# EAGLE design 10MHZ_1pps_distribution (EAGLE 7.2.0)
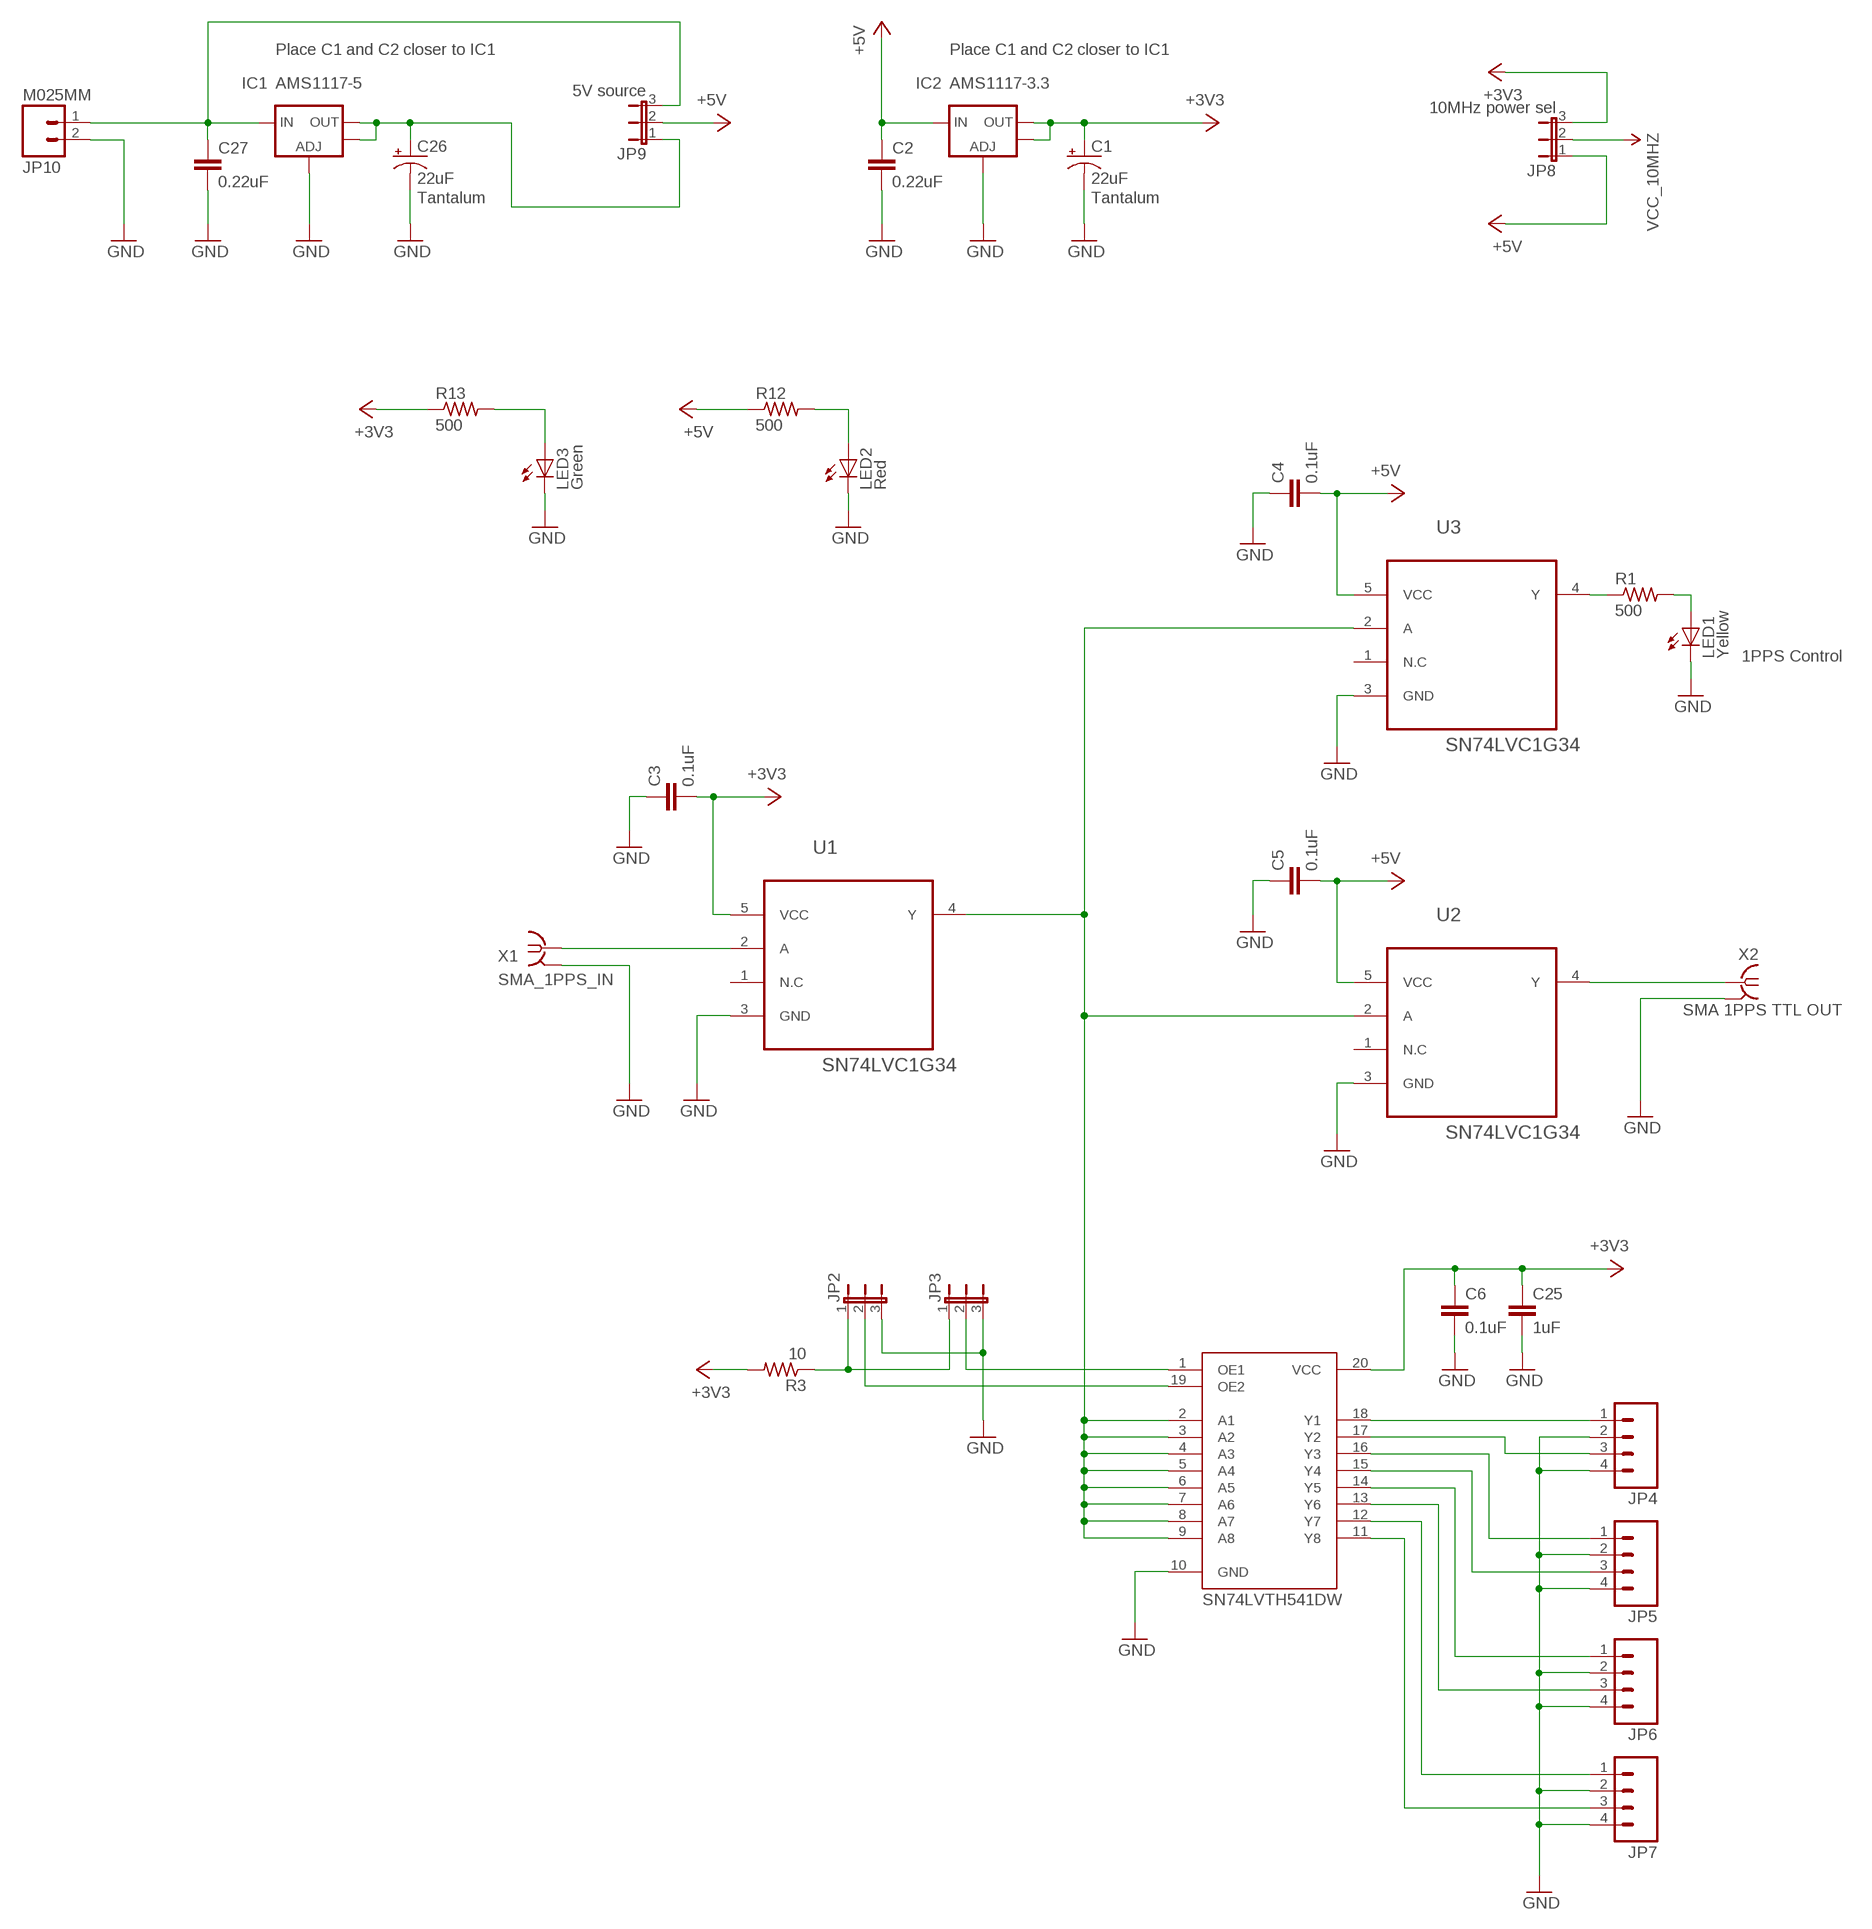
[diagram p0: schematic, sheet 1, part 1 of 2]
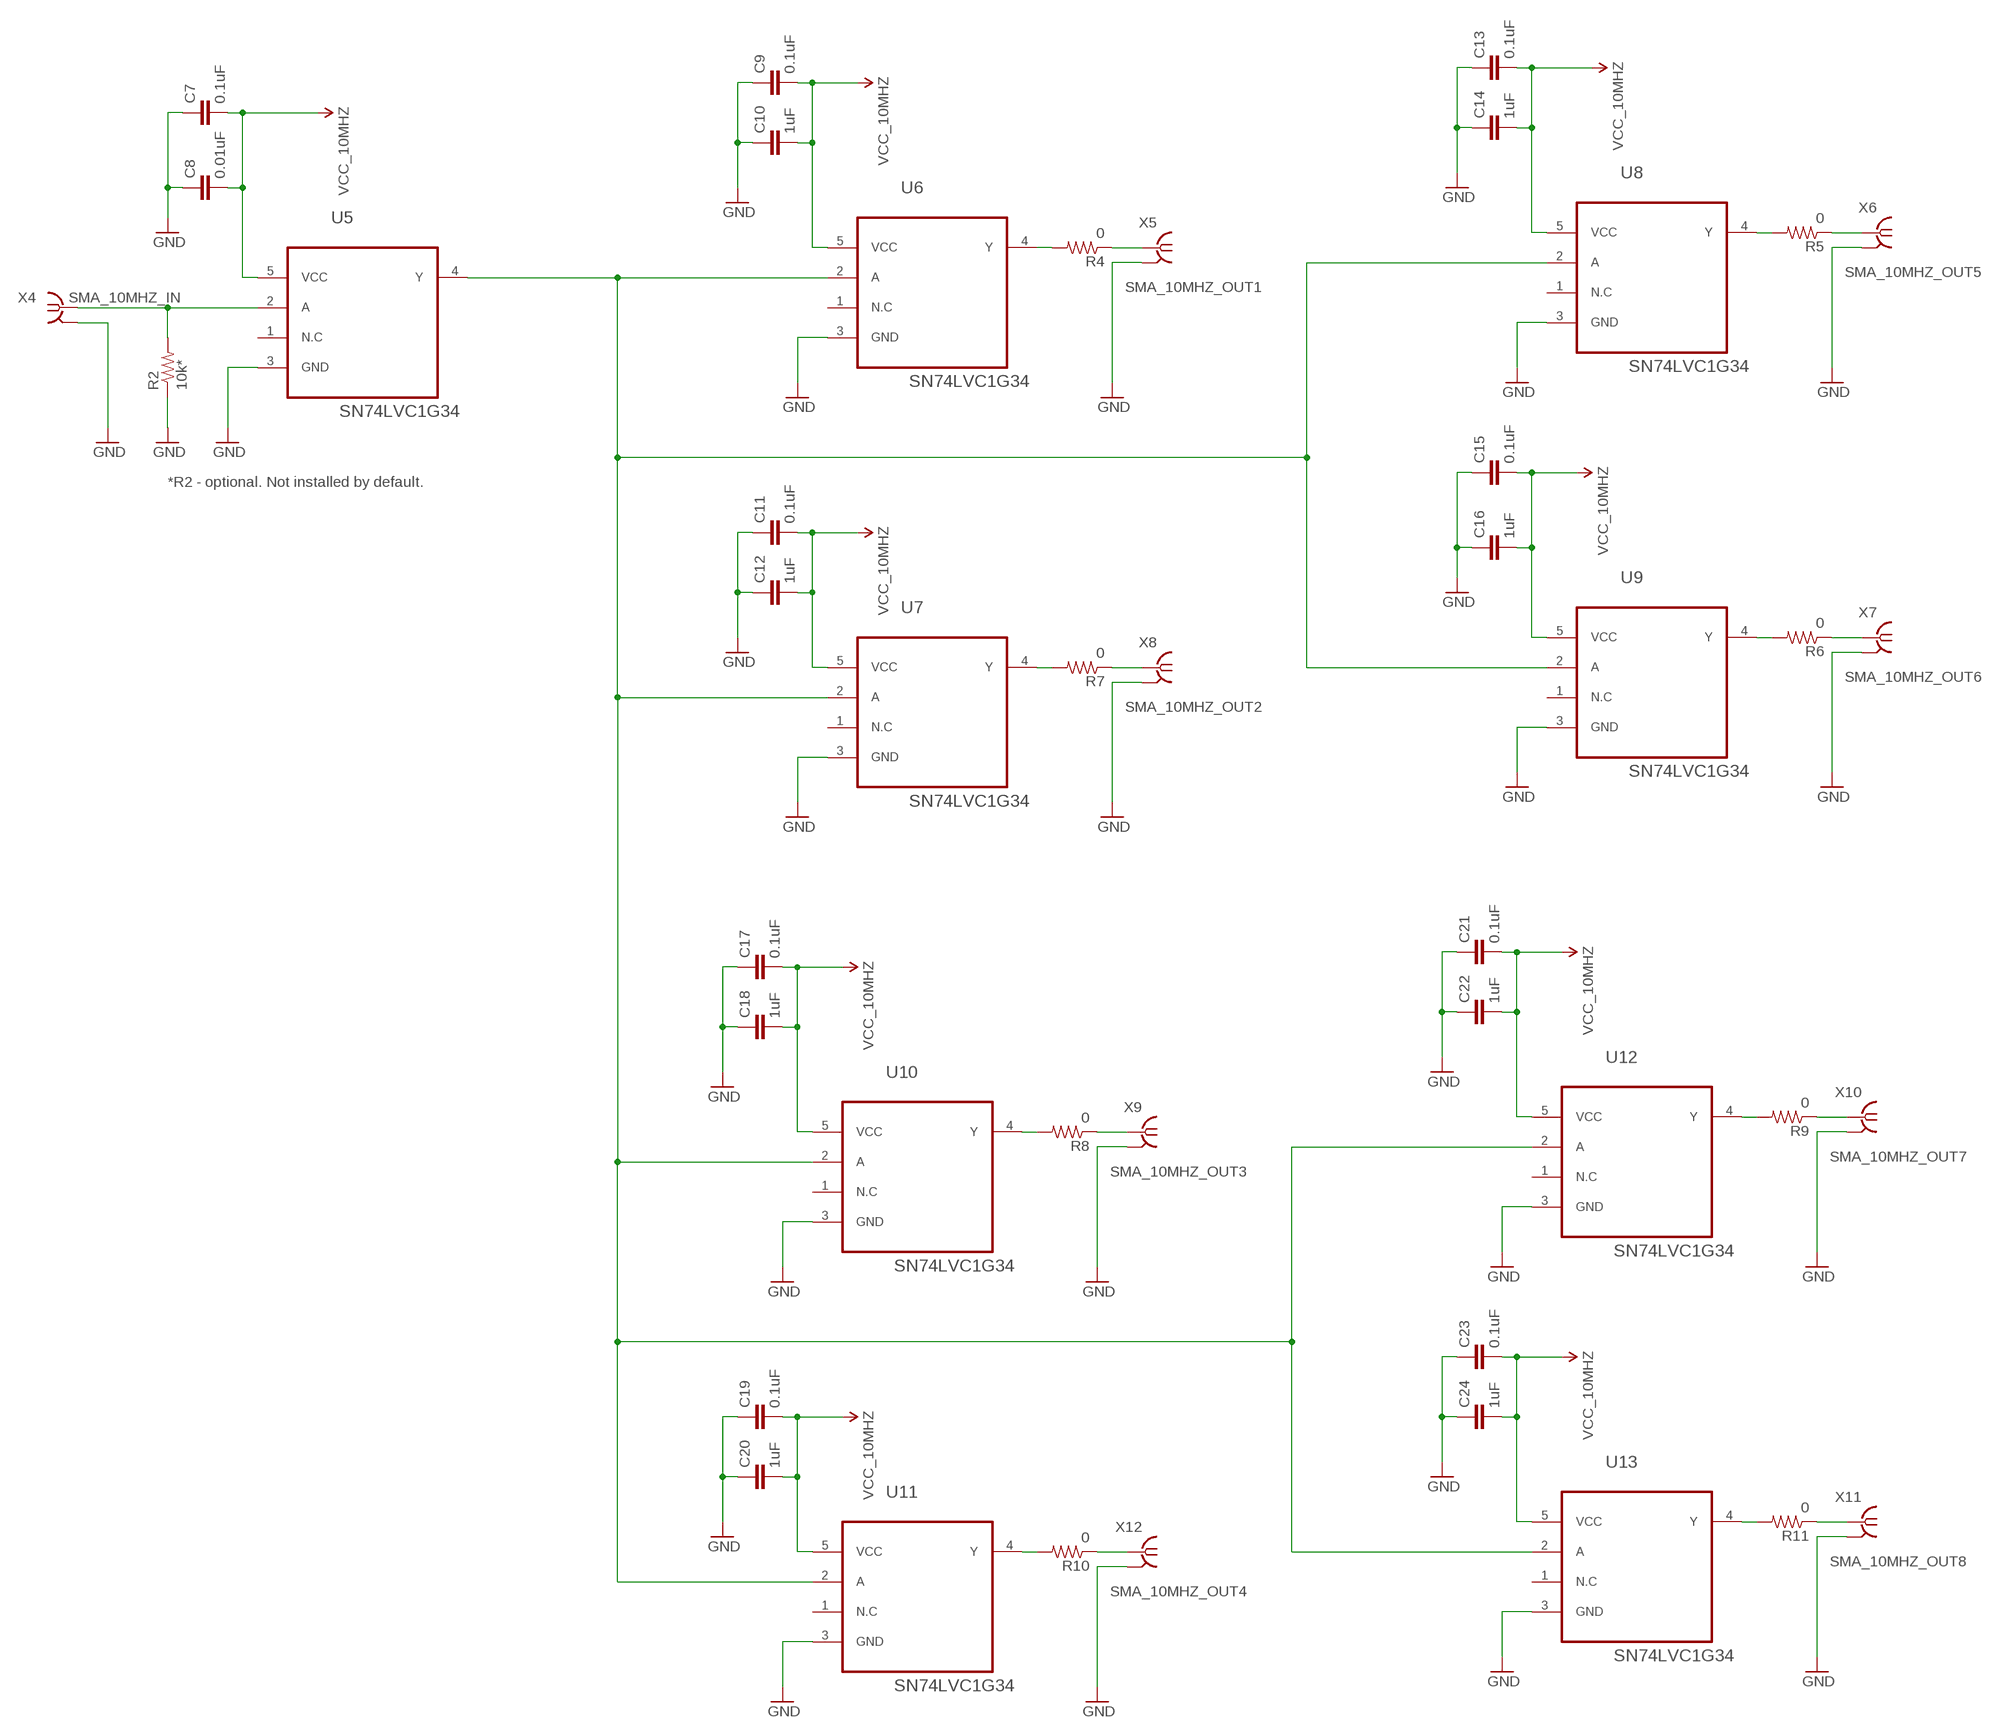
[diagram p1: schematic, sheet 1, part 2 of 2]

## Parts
C1  22uF  CPOL-USD/7343-31W  [D/7343-31W]
C2  0.22uF  C-EUC0805  [C0805]
C3  0.1uF  C-EUC0805  [C0805]
C4  0.1uF  C-EUC0805  [C0805]
C5  0.1uF  C-EUC0805  [C0805]
C6  0.1uF  C-EUC0805  [C0805]
C7  0.1uF  C-EUC0805  [C0805]
C8  0.01uF  C-EUC0805  [C0805]
C9  0.1uF  C-EUC0805  [C0805]
C10  1uF  C-EUC0805  [C0805]
C11  0.1uF  C-EUC0805  [C0805]
C12  1uF  C-EUC0805  [C0805]
C13  0.1uF  C-EUC0805  [C0805]
C14  1uF  C-EUC0805  [C0805]
C15  0.1uF  C-EUC0805  [C0805]
C16  1uF  C-EUC0805  [C0805]
C17  0.1uF  C-EUC0805  [C0805]
C18  1uF  C-EUC0805  [C0805]
C19  0.1uF  C-EUC0805  [C0805]
C20  1uF  C-EUC0805  [C0805]
C21  0.1uF  C-EUC0805  [C0805]
C22  1uF  C-EUC0805  [C0805]
C23  0.1uF  C-EUC0805  [C0805]
C24  1uF  C-EUC0805  [C0805]
C25  1uF  C-EUC0805  [C0805]
C26  22uF  CPOL-USD/7343-31W  [D/7343-31W]
C27  0.22uF  C-EUC0805  [C0805]
IC1  AMS1117-5  LD117AS12TR  [SOT223]
IC2  AMS1117-3.3  LD117AS12TR  [SOT223]
JP2  JP2E  [JP2]
JP3  JP2E  [JP2]
JP4  M04LOCK  [1X04_LOCK]
JP5  M04LOCK  [1X04_LOCK]
JP6  M04LOCK  [1X04_LOCK]
JP7  M04LOCK  [1X04_LOCK]
JP8  10MHz power sel  JP2E  [JP2]
JP9  5V source  JP2E  [JP2]
JP10  M025MM  [SCREWTERMINAL-5MM-2]
LED1  Yellow  LEDSML0805  [SML0805]
LED2  Red  LEDSML0805  [SML0805]
LED3  Green  LEDSML0805  [SML0805]
R1  500  R-US_R0805  [R0805]
R2  10k*  R-US_R0805  [R0805]
R3  10  R-US_R0805  [R0805]
R4  0  R-US_R0805  [R0805]
R5  0  R-US_R0805  [R0805]
R6  0  R-US_R0805  [R0805]
R7  0  R-US_R0805  [R0805]
R8  0  R-US_R0805  [R0805]
R9  0  R-US_R0805  [R0805]
R10  0  R-US_R0805  [R0805]
R11  0  R-US_R0805  [R0805]
R12  500  R-US_R0805  [R0805]
R13  500  R-US_R0805  [R0805]
U1  SN74LVC1G34  SN74LVC1G07DCK6  [SOT65P210X110-5N]
U2  SN74LVC1G34  SN74LVC1G07DCK6  [SOT65P210X110-5N]
U3  SN74LVC1G34  SN74LVC1G07DCK6  [SOT65P210X110-5N]
U4  SN74LVTH541DW  [SOIC127P1030X265-20N]
U5  SN74LVC1G34  SN74LVC1G07DCK6  [SOT65P210X110-5N]
U6  SN74LVC1G34  SN74LVC1G07DCK6  [SOT65P210X110-5N]
U7  SN74LVC1G34  SN74LVC1G07DCK6  [SOT65P210X110-5N]
U8  SN74LVC1G34  SN74LVC1G07DCK6  [SOT65P210X110-5N]
U9  SN74LVC1G34  SN74LVC1G07DCK6  [SOT65P210X110-5N]
U10  SN74LVC1G34  SN74LVC1G07DCK6  [SOT65P210X110-5N]
U11  SN74LVC1G34  SN74LVC1G07DCK6  [SOT65P210X110-5N]
U12  SN74LVC1G34  SN74LVC1G07DCK6  [SOT65P210X110-5N]
U13  SN74LVC1G34  SN74LVC1G07DCK6  [SOT65P210X110-5N]
X1  SMA_1PPS_IN  SMA-142-0701-801/806  [J502-ND-142-0701-801/806]
X2  SMA 1PPS TTL OUT  SMA-142-0701-801/806  [J502-ND-142-0701-801/806]
X4  SMA_10MHZ_IN  SMA-142-0701-801/806  [J502-ND-142-0701-801/806]
X5  SMA_10MHZ_OUT1  SMA-142-0701-801/806  [J502-ND-142-0701-801/806]
X6  SMA_10MHZ_OUT5  SMA-142-0701-801/806  [J502-ND-142-0701-801/806]
X7  SMA_10MHZ_OUT6  SMA-142-0701-801/806  [J502-ND-142-0701-801/806]
X8  SMA_10MHZ_OUT2  SMA-142-0701-801/806  [J502-ND-142-0701-801/806]
X9  SMA_10MHZ_OUT3  SMA-142-0701-801/806  [J502-ND-142-0701-801/806]
X10  SMA_10MHZ_OUT7  SMA-142-0701-801/806  [J502-ND-142-0701-801/806]
X11  SMA_10MHZ_OUT8  SMA-142-0701-801/806  [J502-ND-142-0701-801/806]
X12  SMA_10MHZ_OUT4  SMA-142-0701-801/806  [J502-ND-142-0701-801/806]

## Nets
10MHZ_ROUTE1: U5.4(Y) U6.2(A) U7.2(A) U8.2(A) U9.2(A) U10.2(A) U11.2(A) U12.2(A) U13.2(A)
+3V3: C1.+ C3.2 C6.1 C25.1 IC2.2(OUT) IC2.4(OUT1) JP8.3 R3.2 R13.1 U1.5(VCC) U4.20(VCC)
+5V: C2.1 C4.2 C5.2 IC2.3(IN) JP8.1 JP9.2 R12.1 U2.5(VCC) U3.5(VCC)
GND: C1.- C2.2 C3.1 C4.1 C5.1 C6.2 C7.1 C8.1 C9.1 C10.1 C11.1 C12.1 C13.1 C14.1 C15.1 C16.1 C17.1 C18.1 C19.1 C20.1 C21.1 C22.1 C23.1 C24.1 C25.2 C26.- C27.2 IC1.1(ADJ) IC2.1(ADJ) JP2.3 JP3.3 JP4.2 JP4.4 JP5.2 JP5.4 JP6.2 JP6.4 JP7.2 JP7.4 JP10.2 LED1.C LED2.C LED3.C R2.1 U1.3(GND) U2.3(GND) U3.3(GND) U4.10(GND) U5.3(GND) U6.3(GND) U7.3(GND) U8.3(GND) U9.3(GND) U10.3(GND) U11.3(GND) U12.3(GND) U13.3(GND) X1.G@1(GND) X2.G@1(GND) X4.G@1(GND) X5.G@1(GND) X6.G@1(GND) X7.G@1(GND) X8.G@1(GND) X9.G@1(GND) X10.G@1(GND) X11.G@1(GND) X12.G@1(GND)
N$1: U1.2(A) X1.1
N$2: R1.1 U3.4(Y)
N$3: LED1.A R1.2
N$4: U1.4(Y) U2.2(A) U3.2(A) U4.2(A1) U4.3(A2) U4.4(A3) U4.5(A4) U4.6(A5) U4.7(A6) U4.8(A7) U4.9(A8)
N$5: U2.4(Y) X2.1
N$6: JP3.2 U4.1(OE1)
N$7: JP2.2 U4.19(OE2)
N$8: LED2.A R12.2
N$9: LED3.A R13.2
N$10: JP2.1 JP3.1 R3.1
N$14: R2.2 U5.2(A) X4.1
N$15: R8.2 U10.4(Y)
N$16: R10.2 U11.4(Y)
N$17: R4.1 X5.1
N$18: R9.2 U12.4(Y)
N$19: R7.2 U7.4(Y)
N$20: R11.2 U13.4(Y)
N$21: R5.2 U8.4(Y)
N$23: R6.2 U9.4(Y)
N$27: C27.1 IC1.3(IN) JP9.3 JP10.1
N$28: R4.2 U6.4(Y)
N$29: C26.+ IC1.2(OUT) IC1.4(OUT1) JP9.1
N$30: R5.1 X6.1
N$31: R7.1 X8.1
N$32: R6.1 X7.1
N$33: R8.1 X9.1
N$34: R9.1 X10.1
N$35: R10.1 X12.1
N$36: R11.1 X11.1
PPS_OUT_Y1: JP4.1 U4.18(Y1)
PPS_OUT_Y2: JP4.3 U4.17(Y2)
PPS_OUT_Y3: JP5.1 U4.16(Y3)
PPS_OUT_Y4: JP5.3 U4.15(Y4)
PPS_OUT_Y5: JP6.1 U4.14(Y5)
PPS_OUT_Y6: JP6.3 U4.13(Y6)
PPS_OUT_Y7: JP7.1 U4.12(Y7)
PPS_OUT_Y8: JP7.3 U4.11(Y8)
VCC_10MHZ: C7.2 C8.2 C9.2 C10.2 C11.2 C12.2 C13.2 C14.2 C15.2 C16.2 C17.2 C18.2 C19.2 C20.2 C21.2 C22.2 C23.2 C24.2 JP8.2 U5.5(VCC) U6.5(VCC) U7.5(VCC) U8.5(VCC) U9.5(VCC) U10.5(VCC) U11.5(VCC) U12.5(VCC) U13.5(VCC)
Unconnected: U1.1(N.C) U2.1(N.C) U3.1(N.C) U5.1(N.C) U6.1(N.C) U7.1(N.C) U8.1(N.C) U9.1(N.C) U10.1(N.C) U11.1(N.C) U12.1(N.C) U13.1(N.C)

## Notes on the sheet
- Place C1 and C2 closer to IC1 | Place C1 and C2 closer to IC1
- Tantalum | Tantalum
- *R2 - optional. Not installed by default.
- 1PPS Control

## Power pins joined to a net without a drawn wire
GND: X1.G@2(GND) X1.G@3(GND) X1.G@4(GND) X2.G@2(GND) X2.G@3(GND) X2.G@4(GND) X4.G@2(GND) X4.G@3(GND) X4.G@4(GND) X5.G@2(GND) X5.G@3(GND) X5.G@4(GND) X6.G@2(GND) X6.G@3(GND) X6.G@4(GND) X7.G@2(GND) X7.G@3(GND) X7.G@4(GND) X8.G@2(GND) X8.G@3(GND) X8.G@4(GND) X9.G@2(GND) X9.G@3(GND) X9.G@4(GND) X10.G@2(GND) X10.G@3(GND) X10.G@4(GND) X11.G@2(GND) X11.G@3(GND) X11.G@4(GND) X12.G@2(GND) X12.G@3(GND) X12.G@4(GND)

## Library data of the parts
C1 C26 = resistor:CPOL-US: POLARIZED CAPACITOR, American symbol
C2-C25 C27 = resistor:C-EU: CAPACITOR, European symbol
IC1 IC2 = v-reg:LD117A?*: Low drop fixed and adjustable positive voltage regulators 1 A Source: http://www.st.com/stonline/products/literature/ds/7194/ld1117axx.pdf
JP2 JP3 JP8 JP9 = jumper:JP2E: JUMPER
JP4-JP7 = SparkFun-Connectors:M04: Header 4 Standard 4-pin 0.1" header. Use with straight break away headers (SKU : PRT-00116), right angle break away headers (PRT-00553), swiss pins (PRT-00743), machine pins (PRT-00117), and female headers (PRT-00115). Molex polarized connector foot print use with SKU : PRT-08231 with associated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
JP10 = SparkFun-Connectors:M02: Standard 2-pin 0.1" header. Use with
LED1-LED3 = led:LED: LED
R1 R12 R13 = rcl:R-US_: RESISTOR, American symbol
R2-R11 = adafruit:R-US_: RESISTOR, American symbol
U1-U3 U5-U13 = Texas Instruments_By_element14_Batch_1:SN74LVC1G07DCK6: BUFFER; MPN: SN74LVC1G07DCK6; OC_FARNELL: 1236609; OC_NEWARK: 13M2906; PACKAGE: SC-70-5; SUPPLIER: Texas Instruments
U4 = Texas Instruments_By_element14_Batch_1:SN74LVTH541DW: ABT OCTAL buffer/driver with 3-state outputs; MPN: SN74LVTH541DW; PACKAGE: SOIC-20; SUPPLIER: Texas Instruments
X1 X2 X4-X12 = con-coax:SMA-: SMA 50 Ohm End Launch Jack Receptacle - Round Contact Johnson Components Source: www.johnsoncomponents.com .. J502-ND.pdf

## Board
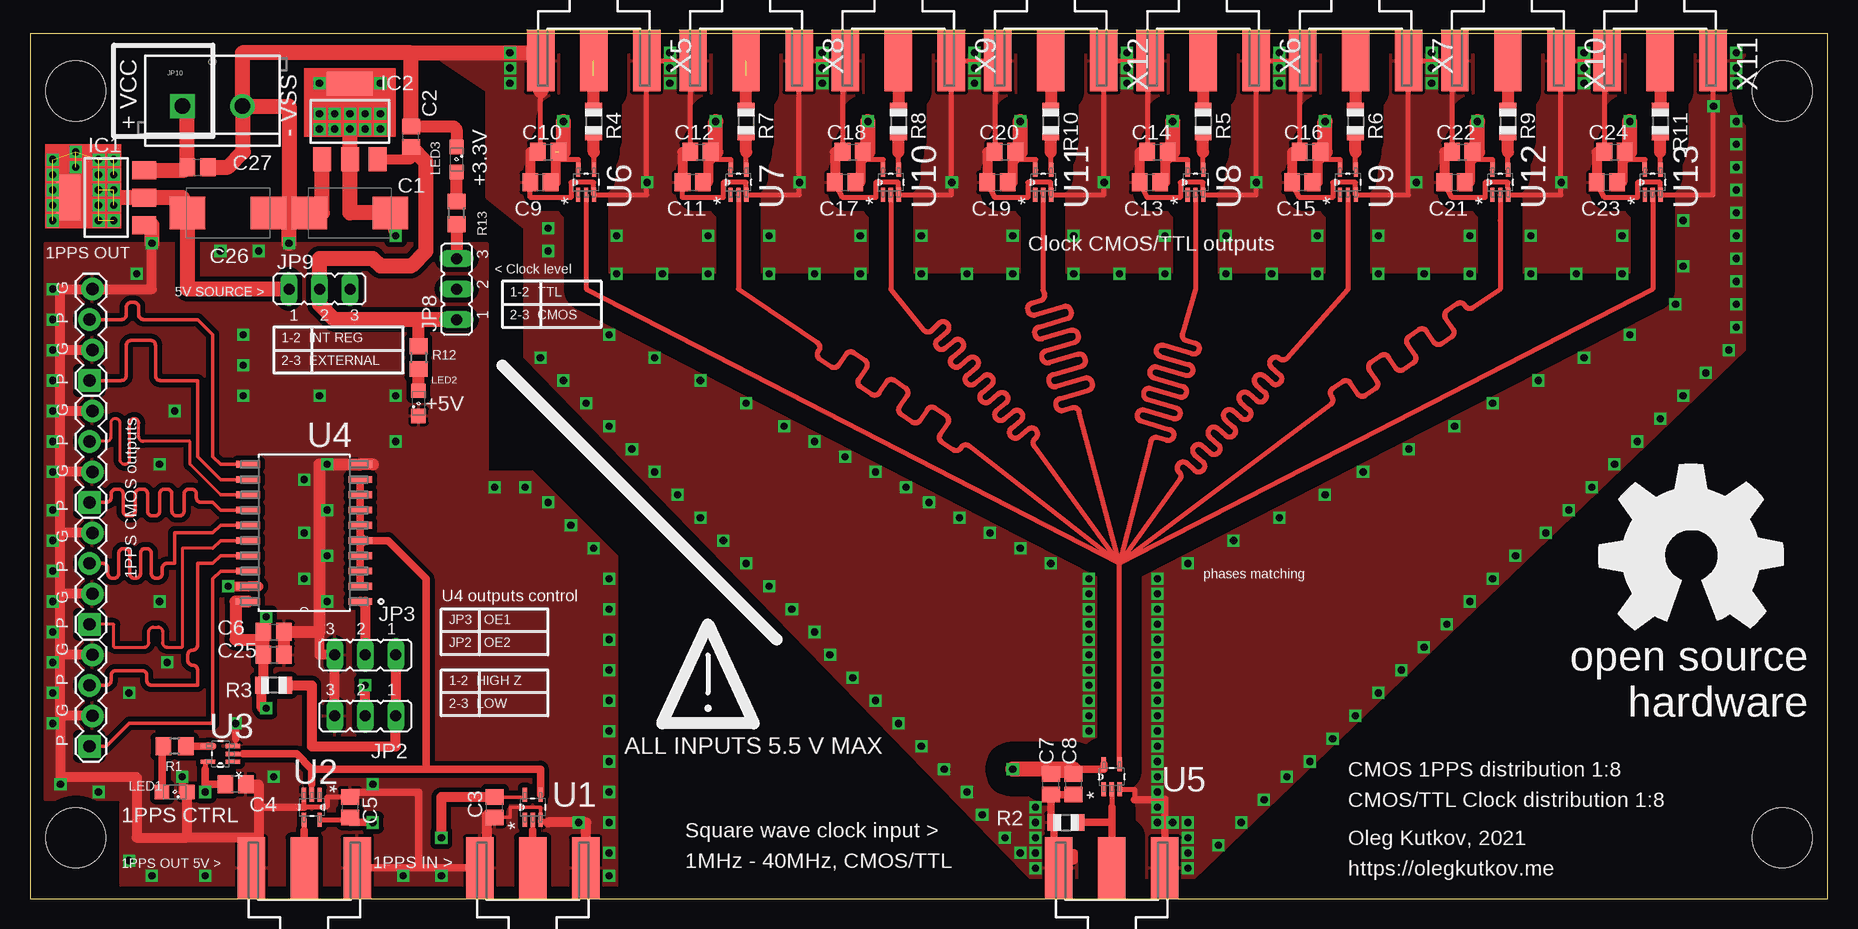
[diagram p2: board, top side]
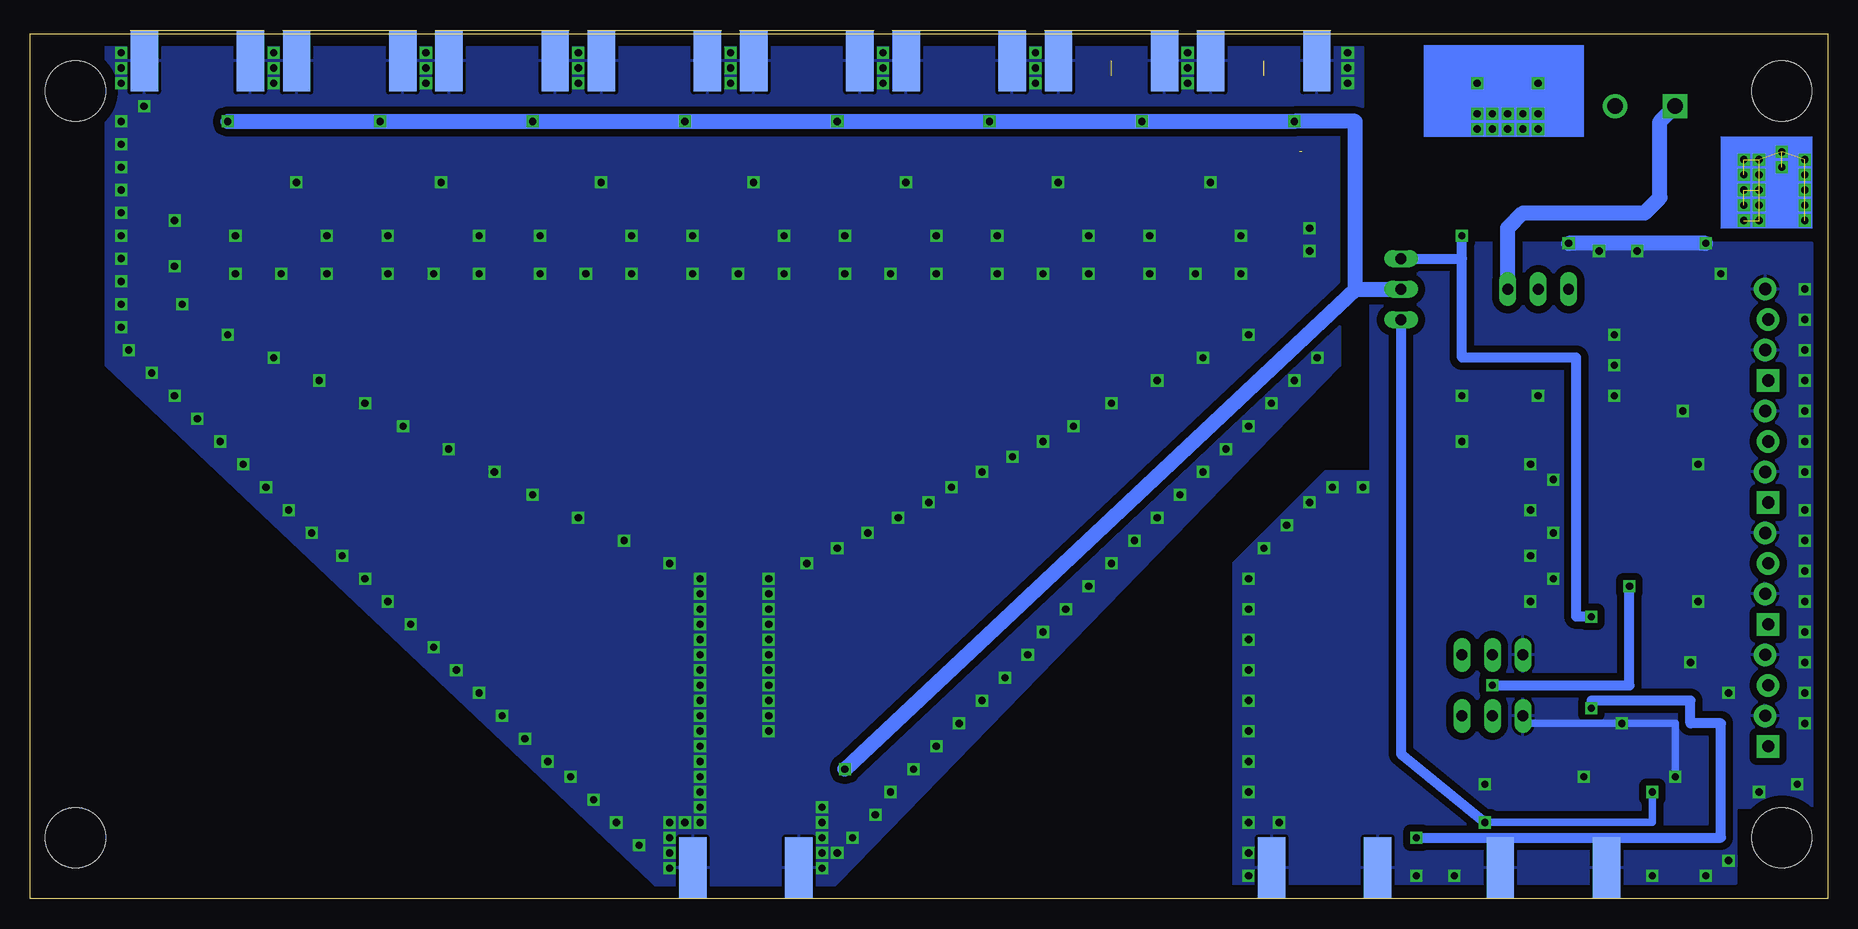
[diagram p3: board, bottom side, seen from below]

Size 149.84 x 72.39 mm. Coordinates in mm from the lower left corner, seen from the top.
Outline: 0,0 149.84,0 149.84,72.06 0,72.06 0,0
Copper layers (1*16): Top 0.035mm / dielectric 1.5mm / Bottom 0.035mm
Design rules "default": minimum track width 10mil, minimum drill 24mil, track to track 8mil, track to pad 8mil, pad to pad 8mil, via to via 8mil, smd to smd 8mil, copper to edge 40mil, drill to drill 8mil, minimum pad ring 10mil, minimum via ring 8mil, stop-mask expansion 4mil, vias tented up to drill 0mil, thermal gap 10mil
Holes 5 mm at 3.81,67.31 146.05,67.31 146.05,5.08 3.81,5.08

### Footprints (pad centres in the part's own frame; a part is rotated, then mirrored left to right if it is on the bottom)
D/7343-31W = smd 2.95 x 2.7: + 3.375,0; - -3.375,0
C0805 = smd 1.3 x 1.5: 1 -0.85,0; 2 0.85,0
SOT223 = smd 1.5 x 2: 1 -2.3,-3.15; 2 0,-3.15; 3 2.3,-3.15 | smd 3.8 x 2: 4 0,3.15
JP2 = drill 0.914 long: 1 -2.54,0; 2 0,0; 3 2.54,0
1X04_LOCK = drill 1.016 pad 1.88 square: 1 0,0.127 | drill 1.016 pad 1.88: 2 2.54,-0.127; 3 5.08,0.127; 4 7.62,-0.127
SCREWTERMINAL-5MM-2 = drill 1.3 pad 2.032 square: 1 0,0 | drill 1.3 pad 2.032: 2 5,0
SML0805 = smd 1.2 x 1.2: A 1.05,0; C -1.05,0
R0805 = smd 1.3 x 1.5: 1 -0.95,0; 2 0.95,0
R0805' = smd 1.1 x 1.4: 1 -1,0; 2 1,0
SOT65P210X110-5N = smd 1.168 x 0.356: 1 -1.041,0.66; 2 -1.041,0; 3 -1.041,-0.66; 4 1.041,-0.66; 5 1.041,0.66
SOIC127P1030X265-20N = smd 1.981 x 0.559: 1 -4.674,5.715; 2 -4.674,4.445; 3 -4.674,3.175; 4 -4.674,1.905; 5 -4.674,0.635; 6 -4.674,-0.635; 7 -4.674,-1.905; 8 -4.674,-3.175; 9 -4.674,-4.445; 10 -4.674,-5.715; 11 4.674,-5.715; 12 4.674,-4.445; 13 4.674,-3.175; 14 4.674,-1.905; 15 4.674,-0.635; 16 4.674,0.635; 17 4.674,1.905; 18 4.674,3.175; 19 4.674,4.445; 20 4.674,5.715
J502-ND-142-0701-801/806 = smd 5.08 x 2.286: 1 2.565,0; G@1 2.565,4.42; G@2 2.565,-4.42 | smd 5.08 x 2.286 bottom: G@3 2.565,4.42; G@4 2.565,-4.42

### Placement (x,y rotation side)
C1  26.67,57.15 0 top
C2  31.75,63.5 90 top
C3  38.73,7.62 90 top
C4  17.14,9.53 180 top
C5  26.67,7.62 270 top
C6  20.32,22.22 0 top
C7  85.09,9.53 90 top
C8  87,9.53 90 top
C9  42.55,59.69 0 top
C10  43.18,62.23 0 top
C11  55.24,59.69 0 top
C12  55.88,62.23 0 top
C13  93.34,59.69 0 top
C14  93.98,62.23 0 top
C15  106.05,59.69 0 top
C16  106.68,62.23 0 top
C17  67.94,59.69 0 top
C18  68.58,62.23 0 top
C19  80.64,59.69 0 top
C20  81.28,62.23 0 top
C21  118.75,59.69 0 top
C22  119.38,62.23 0 top
C23  131.44,59.69 0 top
C24  132.08,62.23 0 top
C25  20.32,20.32 0 top
C26  16.51,57.15 180 top
C27  13.97,60.96 0 top
IC1  6.35,58.42 90 top
IC2  26.67,64.77 0 top
JP2  27.94,15.24 180 top
JP3  27.94,20.32 180 top
JP4  5.08,12.7 90 top
JP5  5.08,22.86 90 top
JP6  5.08,33.02 90 top
JP7  5.08,43.18 90 top
JP8  35.56,50.8 90 top
JP9  24.13,50.8 0 top
JP10  12.7,66.04 0 top
LED1  12.06,8.89 180 top
LED2  32.38,41.28 90 top
LED3  35.56,61.59 270 top
R1  12.06,12.7 180 top
R2  10k*  [R0805']  86.36,6.35 0 top
R3  10  [R0805']  20.32,17.78 180 top
R4  0  [R0805']  46.99,64.77 270 top
R5  0  [R0805']  97.79,64.77 270 top
R6  0  [R0805']  110.49,64.77 270 top
R7  0  [R0805']  59.69,64.77 270 top
R8  0  [R0805']  72.39,64.77 270 top
R9  0  [R0805']  123.19,64.77 270 top
R10  0  [R0805']  85.09,64.77 270 top
R11  0  [R0805']  135.89,64.77 270 top
R12  32.38,45.09 270 top
R13  35.56,57.15 90 top
U1  41.91,7.62 90 top
U2  23.5,7.62 270 top
U3  15.88,12.07 180 top
U4  22.86,30.48 180 top
U5  90.17,10.16 90 top
U6  46.35,59.69 90 top
U7  59.05,59.69 90 top
U8  97.16,59.69 90 top
U9  109.86,59.69 90 top
U10  71.75,59.69 90 top
U11  84.45,59.69 90 top
U12  122.56,59.69 90 top
U13  135.25,59.69 90 top
U$1  [OSHW_16MM]  138.43,28.57 0 top
X1  41.91,0 90 top
X2  22.86,0 90 top
X4  90.17,0 90 top
X5  46.99,72.39 270 top
X6  97.79,72.39 270 top
X7  110.49,72.39 270 top
X8  59.69,72.39 270 top
X9  72.39,72.39 270 top
X10  123.19,72.39 270 top
X11  135.89,72.39 270 top
X12  85.09,72.39 270 top

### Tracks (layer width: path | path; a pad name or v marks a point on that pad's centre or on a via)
10MHZ_ROUTE1
  Top 0.406: U5.4 90.81,11.2 90.81,27.94 | U13.2 135.25,50.8 90.81,27.94 | U10.2 71.75,50.8 74.5,47.38 arc90 75.15,47.32 75.82,47.99 arc-90 76.47,47.93 76.5,47.89 arc-90 76.44,47.25 75.66,46.59 arc90 75.6,45.95 75.63,45.91 arc90 76.27,45.86 77.05,46.51 arc-90 77.7,46.45 77.73,46.41 arc-90 77.67,45.77 76.89,45.12 arc90 76.83,44.47 76.86,44.44 arc90 77.5,44.38 78.28,45.03 arc-90 78.93,44.97 78.96,44.94 arc-90 78.9,44.29 78.12,43.64 arc90 78.06,43 78.09,42.96 arc90 78.73,42.9 79.52,43.55 arc-90 80.16,43.49 80.19,43.46 arc-90 80.13,42.81 79.35,42.16 arc90 79.29,41.52 79.32,41.48 arc90 79.96,41.42 80.75,42.08 arc-90 81.39,42.02 81.42,41.98 arc-90 81.36,41.34 80.58,40.68 arc90 80.52,40.04 80.55,40 arc90 81.19,39.95 81.98,40.6 arc-90 82.62,40.54 82.65,40.5 arc-90 82.59,39.86 81.81,39.21 arc90 81.75,38.56 81.78,38.53 arc90 82.43,38.47 83.21,39.12 arc-90 83.85,39.06 83.89,39.03 arc-90 83.83,38.38 83.78,38.35 arc90 83.73,37.7 90.81,27.94 | U8.2 97.16,50.8 96.06,47.09 arc90 96.37,46.52 97.14,46.3 arc-90 97.45,45.73 97.44,45.71 arc-90 96.88,45.4 94.47,46.11 arc90 93.9,45.8 93.89,45.77 arc90 94.2,45.2 96.61,44.5 arc-90 96.92,43.93 96.91,43.91 arc-90 96.35,43.6 93.94,44.31 arc90 93.37,44 93.36,43.97 arc90 93.67,43.41 96.08,42.7 arc-90 96.39,42.13 96.38,42.11 arc-90 95.82,41.8 93.41,42.51 arc90 92.84,42.2 92.83,42.17 arc90 93.14,41.61 95.55,40.9 arc-90 95.86,40.33 95.86,40.31 arc-90 95.29,40 92.88,40.71 arc90 92.31,40.4 92.3,40.38 arc90 92.61,39.81 95.02,39.1 arc-90 95.33,38.53 95.33,38.51 arc-90 94.76,38.2 93.99,38.42 arc90 93.42,38.11 90.81,27.94
  Top 0.406: U9.2 109.86,50.8 104.78,45.05 arc-90 104.13,45.01 104.13,45.01 arc90 103.48,44.97 103.44,44.93 arc90 103.48,44.29 104.19,43.67 arc-90 104.22,43.02 104.19,42.98 arc-90 103.54,42.94 102.84,43.56 arc90 102.2,43.52 102.16,43.48 arc90 102.2,42.83 102.9,42.21 arc-90 102.94,41.57 102.9,41.53 arc-90 102.26,41.48 101.56,42.1 arc90 100.91,42.06 100.88,42.02 arc90 100.92,41.38 101.62,40.76 arc-90 101.66,40.11 101.62,40.07 arc-90 100.97,40.03 100.27,40.65 arc90 99.63,40.61 99.59,40.56 arc90 99.63,39.92 100.33,39.3 arc-90 100.37,38.66 100.33,38.61 arc-90 99.69,38.57 98.99,39.19 arc90 98.34,39.15 98.31,39.11 arc90 98.35,38.46 99.05,37.85 arc-90 99.09,37.2 99.05,37.16 arc-90 98.41,37.12 97.7,37.74 arc90 97.06,37.7 97.02,37.65 arc90 97.06,37.01 97.76,36.39 arc-90 97.8,35.75 97.77,35.7 arc-90 97.12,35.66 96.42,36.28 arc90 95.78,36.24 95.74,36.2 arc90 95.78,35.55 95.79,35.55 arc-90 95.83,34.9 90.81,27.94 | U6.2 46.35,50.8 90.81,27.94 | 59.05,59.06 U7.2 59.05,50.8 65.64,46.32 arc-90 65.76,45.69 65.7,45.61 arc90 65.83,44.97 66.77,44.33 arc90 67.4,44.45 68.02,45.37 arc-90 68.66,45.49 69.6,44.85 arc-90 69.72,44.22 69.09,43.3 arc90 69.22,42.67 70.16,42.03 arc90 70.79,42.15 71.41,43.07 arc-90 72.05,43.19 72.99,42.55 arc-90 73.11,41.91 72.49,41 arc90 72.61,40.36 73.55,39.72 arc90 74.18,39.84 74.81,40.76 arc-90 75.44,40.88 76.38,40.24 arc-90 76.5,39.61 75.88,38.69 arc90 76,38.06 76.94,37.42 arc90 77.57,37.54 77.63,37.62 arc-90 78.26,37.74 90.81,27.94 | 122.56,56.52 U12.2 122.56,50.8 120.28,49.25 arc-90 119.64,49.37 119.59,49.45 arc90 118.95,49.57 118.12,49.01 arc90 118,48.37 118.62,47.46 arc-90 118.5,46.82 117.67,46.25 arc-90 117.03,46.38 116.41,47.29 arc90 115.78,47.41 114.94,46.85 arc90 114.82,46.21 115.44,45.3 arc-90 115.32,44.66 114.49,44.09 arc-90 113.86,44.21 113.23,45.13 arc90 112.6,45.25 111.77,44.69 arc90 111.64,44.05 112.27,43.13 arc-90 112.15,42.5 111.31,41.93 arc-90 110.68,42.05 110.06,42.97 arc90 109.42,43.09 108.59,42.53 arc90 108.47,41.89 108.52,41.81 arc-90 108.4,41.17 90.81,27.94
  Top 0.406: 90.81,27.94 87.46,40.59 arc90 86.89,40.9 86.12,40.68 arc-90 85.56,40.99 85.52,41.11 arc-90 85.83,41.67 88.24,42.38 arc90 88.55,42.95 88.52,43.07 arc90 87.95,43.38 85.54,42.67 arc-90 84.97,42.98 84.94,43.09 arc-90 85.25,43.66 87.66,44.37 arc90 87.97,44.94 87.93,45.06 arc90 87.36,45.37 84.95,44.66 arc-90 84.39,44.97 84.35,45.08 arc-90 84.66,45.65 87.07,46.36 arc90 87.38,46.93 87.34,47.04 arc90 86.78,47.35 84.37,46.64 arc-90 83.8,46.95 83.77,47.07 arc-90 84.08,47.64 86.48,48.35 arc90 86.8,48.92 86.76,49.03 arc90 86.19,49.34 83.78,48.63 arc-90 83.22,48.94 83.18,49.06 arc-90 83.49,49.63 84.26,49.85 arc90 84.57,50.42 84.45,50.8 U11.2 84.45,59.06 | 90.81,27.94 90.81,28.57
+3V3  (via drill 0.6)
  Top 0.305: C3.2 41.25,8.47 U1.5
  Top 0.61: 17.14,21.59 19.68,21.59 v19.68,23.5
  Top 0.813: 29.84,57.15 v30.48,55.25 30.48,57.15 C1.+ | C25.1 19.47,17.78 R3.2 19.32,15.87 v19.68,15.87 | C3.2 34.29,8.47 v34.29,5.08
  Top 1.016: C25.1 19.47,21.59 | 19.47,21.59 C6.1 | U4.20 17.14,24.76 17.14,21.59 19.47,21.59 | R13.1 JP8.3
  Top 1.27: C1.+ 29.84,57.15 26.67,57.15 IC2.2 v26.67,64.14 v26.67,65.41 IC2.4
  Bottom 0.813: v19.68,23.5 20.95,23.5 20.95,45.09 30.48,45.09 30.48,53.34 | JP8.3 30.48,53.34 | 30.48,53.34 v30.48,55.25 | v34.29,5.08 8.89,5.08 8.89,14.61 11.43,14.61 11.43,16.51 19.68,16.51 v19.68,15.87
+5V  (via drill 0.6)
  Top 0.406: U2.5 26.67,6.58 C5.2 | U3.5 14.83,11.43 14.61,11.43 14.61,10.79
  Top 0.61: 14.61,10.79 14.61,9.53 | 14.61,9.53 v14.61,8.89 | v28.57,6.35 26.67,6.35 C5.2 | C4.2 14.61,9.53
  Top 0.813: IC2.3 31.75,61.62 C2.1
  Top 1.016: R12.1 32.38,48.26
  Top 1.27: JP8.1 32.38,48.26 25.4,48.26 24.13,49.53 JP9.2 24.13,53.34 28.57,53.34 29.21,52.7 31.75,52.7 33.02,53.98 33.02,61.38 C2.1
  Bottom 0.61: v14.61,8.89 14.61,6.35 v28.57,6.35
  Bottom 0.813: JP8.1 35.56,12.07 v28.57,6.35
  other vias: 35.56,48.26
GND  (via drill 0.6)
  Top 0.305: C3.1 40.01,6.77 40.01,7.62 42.57,7.62 U1.3 | U3.3 17.14,12.72 17.14,13.33
  Top 0.406: X11.G@1 140.31,58.65 U13.3 135.89,58.65 135.89,59.69 133.99,59.69 133.99,58.42 131.23,58.42 C23.1 | C10.1 42.57,62.23 42.57,67.31 X5.G@4 | C12.1 55.03,69.83 X8.G@4 55.27,69.85 54.61,69.85 54.61,69.83 X5.G@1 51.41,58.65 U6.3 46.99,58.65 46.99,59.69 45.09,59.69 45.09,58.42 41.7,58.42 C9.1 | C18.1 67.73,69.83 X9.G@4 67.97,69.85 67.31,69.85 67.31,69.83 X8.G@1 64.11,58.65 U7.3 59.69,58.65 59.69,59.69 57.78,59.69 57.78,58.42 54.4,58.42 C11.1 | C20.1 80.43,69.83 X12.G@4 X9.G@1 76.81,58.65 U10.3 72.39,58.65 72.39,59.69 70.48,59.69 70.48,58.42 67.73,58.42 C17.1 | C14.1 93.13,69.83 X6.G@4 X12.G@1 89.51,58.65 U11.3 85.09,58.65 85.09,59.69 83.19,59.69 83.19,58.42 80.43,58.42 C19.1 | C16.1 105.83,69.83 X7.G@4 X6.G@3 102.21,58.65 U8.3 97.79,58.65 97.79,59.69 95.89,59.69 95.89,58.42 93.13,58.42 C13.1 | C22.1 118.53,69.83 X10.G@4 X7.G@1 114.91,58.65 U9.3 110.49,58.65 110.49,59.69 108.58,59.69 108.58,58.42 105.83,58.42 C15.1 | C24.1 131.23,69.83 X11.G@4 X10.G@1 127.61,58.65 U12.3 123.19,59.69 121.28,59.69 121.28,58.42 118.53,58.42 C21.1 | 43.18,6.35 42.57,6.35 U1.3 | C5.1 24.77,8.47 24.77,7.62 22.84,7.62 U2.3 | U5.3 92.08,9.12 92.08,8.25
  Top 0.61: X2.G@4 32.38,2.56 | 32.38,2.56 32.38,8.89 26.67,8.89 C5.1 | 32.38,2.56 X1.G@1 | X2.G@1 19.05,2.56 19.05,5.08 19.05,7.62 | 19.05,7.62 22.84,7.62 | 87.02,3.81 87.02,3.17 | 87.02,3.17 X4.G@1 | X4.G@4 94.61,8.28 93.98,8.25 92.08,8.25 | 19.05,9.53 19.05,7.62 | LED1.C 12.7,8.89 v12.7,10.16 | 17.14,13.33 v17.14,14.61 | 87.02,3.17 85.36,3.17 R2.1 85.09,6.35 C7.1 C8.1
  Top 0.813: 24.13,22.86 24.13,20.32 JP3.3 JP2.3 | X1.G@1 38.1,2.56 38.1,6.98 38.73,6.98 C3.1 | X1.G@4 46.35,2.56 46.35,6.35 43.18,6.35 | 2.54,15.24 2.54,20.32 | JP4.4 2.54,20.32 | 2.54,20.32 2.54,25.4 | JP5.2 2.54,25.4 | 2.54,25.4 2.54,30.48 | JP5.4 2.54,30.48 | 2.54,30.48 2.54,35.56 | JP6.2 2.54,35.56 | 2.54,35.56 2.54,40.64 | JP6.4 2.54,40.64 | 2.54,40.64 2.54,45.72 | JP7.2 2.54,45.72 | 2.54,45.72 2.54,50.8 JP7.4 10.16,50.8 v10.16,54.61 | JP4.2 2.54,15.24 | 2.54,15.24 2.54,10.16 8.89,10.16 8.89,5.08 13.12,5.08 | 13.12,5.08 LED1.C | C4.1 19.05,9.53 19.05,5.08 13.12,5.08 | C10.1 41.7,62.23 C9.1 | C12.1 54.4,62.23 C11.1 | C18.1 67.09,62.23 C17.1 | C20.1 79.8,62.23 C19.1 | C14.1 92.5,62.23 C13.1 | C16.1 105.19,62.23 C15.1 | C22.1 117.89,62.23 C21.1 | C24.1 130.59,62.23 C23.1
  Top 1.016: C25.2 C6.2 24.13,22.22 24.13,22.86 24.13,36.2 U4.10 28.57,36.2 | C2.2 35.34,64.35 35.56,64.14 LED3.C
  Top 1.27: JP10.2 21.59,66.04 21.59,57.15 | 19.68,57.15 C26.- 21.59,57.15 | IC2.1 24.37,57.15 C1.- 21.59,57.15 | IC1.1 10.16,56.12 v10.16,54.61 | v21.59,54.61 21.59,57.15 | C2.2 31.75,70.48 | 31.75,70.48 17.7,70.48 JP10.2 | C27.2 16.51,60.96 17.78,62.23 17.78,65.96 JP10.2 | 31.75,70.48 v40.01,70.48 42.57,70.48 42.57,67.31
  Bottom 0.61: v12.7,10.16 12.7,14.61 v17.14,14.61 25.4,14.61 JP2.3
  Bottom 1.27: v10.16,54.61 v21.59,54.61
  other vias: 8.89,52.07 17.78,46.99 17.78,41.91 24.13,41.91 30.48,41.91 17.78,44.45 38.73,34.29 41.27,34.29 43.18,33.02 45.09,31.11 46.99,29.21 48.26,26.67 48.26,24.13 48.26,21.59 48.26,19.05 48.26,16.51 48.26,13.97 48.26,11.43 48.26,8.89 48.26,6.35 45.72,6.35 48.26,3.81 48.26,1.9 34.29,1.9 31.11,1.9 14.61,1.9 10.16,1.9 8.26,3.17 5.71,8.89 2.54,9.53 1.91,14.61 1.91,17.14 1.91,19.68 1.91,22.22 1.91,24.76 1.91,27.3 1.91,29.84 1.91,32.39 1.91,35.56 1.91,38.1 1.91,40.64 1.91,43.18 1.91,45.72 1.91,48.26 1.91,50.8 30.48,38.1 22.86,34.92 24.77,32.39 22.86,30.48 24.77,28.57 22.86,26.67 24.77,24.76 24.77,36.2 20.32,10.16 28.57,9.53 19.05,53.98 15.88,53.98 40.01,69.22 40.01,67.95 53.34,70.48 53.34,69.22 53.34,67.95 66.04,70.48 66.04,69.22 66.04,67.95 78.74,70.48 78.74,69.22 78.74,67.95 91.44,70.48 91.44,69.22 91.44,67.95 104.14,70.48 104.14,69.22 104.14,67.95 116.84,70.48 116.84,69.22 116.84,67.95 129.54,70.48 129.54,69.22 129.54,67.95 142.24,70.48 142.24,69.22 142.24,67.95 140.34,66.04 142.24,64.77 142.24,62.87 142.24,60.96 142.24,59.06 142.24,57.15 142.24,55.25 142.24,53.34 142.24,51.44 142.24,49.53 142.24,47.62 141.6,45.72 139.7,43.81 137.79,41.91 135.89,40 133.99,38.1 132.08,36.2 130.18,34.29 128.27,32.39 126.36,30.48 123.83,28.57 121.92,26.67 120.02,24.76 118.11,22.86 116.2,20.96 114.3,19.05 112.39,17.14 110.49,15.24 108.58,13.33 106.68,11.43 104.78,10.16 102.87,8.25 100.97,6.35 99.06,4.44 96.52,2.54 96.52,3.81 96.52,5.08 96.52,6.35 95.25,6.35 93.98,6.35 83.82,2.54 83.82,3.81 83.82,5.08 83.82,6.35 83.82,7.62 82.55,3.81 93.98,7.62 93.98,8.89 93.98,10.16 93.98,11.43 93.98,12.7 93.98,13.97 93.98,15.24 93.98,16.51 93.98,17.78 93.98,19.05 93.98,20.32 93.98,21.59 93.98,22.86 93.98,24.13 93.98,25.4 93.98,26.67 12.06,40.64 10.79,36.2 10.79,24.76 11.43,19.68 8.26,17.14 43.18,55.88 43.18,53.98 42.55,45.09 44.45,43.18 46.35,41.28 48.26,39.37 50.16,37.47 52.07,35.56 53.98,33.66 55.88,31.75 57.78,29.84 59.69,27.94 61.59,26.04 63.5,24.13 65.41,22.22 66.67,20.32 68.58,18.41 70.48,16.51 72.39,14.61 74.3,12.7 76.2,10.79 78.11,8.89 79.38,6.98 81.28,5.08 88.27,13.97 88.27,15.24 88.27,16.51 88.27,17.78 88.27,19.05 88.27,20.32 88.27,21.59 88.27,22.86 88.27,24.13 88.27,25.4 88.27,26.67 48.9,52.07 52.7,52.07 56.52,52.07 48.9,55.25 56.52,55.25 61.59,55.25 61.59,52.07 65.41,52.07 69.22,52.07 69.22,55.25 74.3,55.25 74.3,52.07 78.11,52.07 81.92,52.07 81.92,55.25 87,55.25 87,52.07 90.81,52.07 94.61,52.07 94.61,55.25 99.69,55.25 99.69,52.07 103.5,52.07 107.31,52.07 107.31,55.25 112.39,55.25 112.39,52.07 116.2,52.07 120.02,52.07 120.02,55.25 125.09,55.25 125.09,52.07 128.91,52.07 132.72,52.07 132.72,55.25 127.64,59.69 115.57,59.69 102.23,59.69 89.53,59.69 76.83,59.69 64.14,59.69 51.44,59.69 85.09,27.94 82.55,29.21 80.01,30.48 77.47,31.75 74.93,33.02 73.03,34.29 70.48,35.56 67.94,36.83 65.41,38.1 62.87,39.37 59.69,41.28 55.88,43.18 52.07,45.09 48.26,46.99 96.52,27.94 100.33,29.84 104.14,31.75 107.95,33.66 111.12,35.56 114.94,37.47 118.75,39.37 121.92,41.28 125.73,43.18 129.54,45.09 133.35,46.99 137.16,49.53 137.79,52.7 137.79,56.52
  pour Top (isolate 0.406): 1.27,54.61 38.1,54.61 38.1,35.56 41.91,35.56 47.62,29.84 48.9,28.57 48.9,0.63 7.62,0.63 7.62,8.25 1.27,8.25
  pour Bottom (isolate 0.61): 1.27,54.61 38.1,54.61 38.1,35.56 41.91,35.56 49.53,27.94 49.53,1.27 7.62,1.27 7.62,7.62 1.27,7.62
  pour Top (isolate 1.651): 34.29,71.12 41.27,71.75 142.88,71.75 142.88,45.72 95.89,0.63 84.45,0.63 41.27,45.09 41.27,55.88 38.1,58.42 38.1,67.31 34.29,69.85
  pour Bottom (isolate 0.61): 38.73,72.39 143.51,72.39 143.51,44.45 96.52,0 83.82,0 40.64,44.45 40.64,55.88 38.73,58.42
  cutout Top: 48.26,52.07 57.15,52.07 57.15,51.44 48.26,51.44
  cutout Top: 60.96,52.07 69.85,52.07 69.85,51.44 60.96,51.44
  cutout Top: 73.66,52.07 82.55,52.07 82.55,51.44 73.66,51.44
  cutout Top: 86.36,52.07 95.25,52.07 95.25,51.44 86.36,51.44
  cutout Top: 99.06,52.07 107.95,52.07 107.95,51.44 99.06,51.44
  cutout Top: 111.76,52.07 120.65,52.07 120.65,51.44 111.76,51.44
  cutout Top: 124.46,52.07 133.35,52.07 133.35,51.44 124.46,51.44
IC1_HS  (via drill 0.6)  (16 unrouted)
  other vias: 3.81,62.23 3.81,60.96 5.71,56.52 5.71,57.78 5.71,59.06 5.71,60.33 5.71,61.59 6.99,61.59 6.99,60.33 6.99,59.06 6.99,57.78 6.99,56.52 1.91,61.59 1.91,60.33 1.91,59.06 1.91,57.78 1.91,56.52
N$1
  Top 0.305: U1.2 41.91,5.71
  Top 0.61: 41.91,5.71 X1.1
N$2
  Top 0.61: R1.1 14.83,12.7 | 15.24,12.7 14.83,12.7 | 14.83,12.7 U3.4
N$3
  Top 0.61: R1.2 11.02,12.7 LED1.A
N$4
  Top 0.406: U2.2 23.5,9.53 | U3.2 17.78,12.07
  Top 0.61: U1.4 42.55,8.69 42.55,10.79 33.02,10.79 | 23.5,9.53 23.5,10.79 | 23.5,10.79 33.02,10.79 | 17.78,12.07 22.23,12.07 23.5,10.79 | 27.53,30.25 U4.5 | U4.5 27.53,29.44 | U4.5 27.94,29.84 | 27.94,29.84 29.84,29.84 33.02,26.67 33.02,10.79 | U4.9 U4.8 U4.7 U4.6 27.53,30.25 | 27.53,30.25 27.94,29.84 | 27.53,29.44 27.94,29.84 | 27.53,29.44 U4.4 U4.3 U4.2
N$5
  Top 0.406: U2.4 22.86,6.58 22.86,5.71
  Top 0.61: 22.86,5.71 X2.1
N$6
  Top 0.813: U4.1 27.94,24.76 JP3.2
N$7  (via drill 0.6)
  Top 0.813: JP2.2 v27.94,17.78 | v16.51,26.04 U4.19 19.05,26.04
  Bottom 0.813: v27.94,17.78 16.51,17.78 v16.51,26.04
N$8
  Top 1.016: LED2.A R12.2
N$9
  Top 1.016: R13.2 LED3.A
N$10
  Top 0.813: JP3.1 JP2.1 30.48,12.7 23.5,12.7 23.5,17.78 R3.1
N$14
  Top 0.406: U5.2 90.17,7.62
  Top 0.61: 90.17,7.62 90.17,6.35 | 90.17,6.35 X4.1 | R2.2 90.17,6.35
N$15
  Top 0.406: U10.4 72.39,60.73 72.39,62.23
  Top 1.016: 72.39,62.23 R8.2
N$16
  Top 0.406: U11.4 85.09,60.73 85.09,62.23
  Top 1.016: 85.09,62.23 R10.2
N$17  (1 unrouted)
  Top 1.016: R4.1 46.99,68.58
N$18
  Top 0.406: U12.4 123.19,60.73 123.19,62.23
  Top 1.016: 123.19,62.23 R9.2
N$19
  Top 0.406: U7.4 59.69,60.73 59.69,62.23
  Top 1.016: 59.69,62.23 R7.2
N$20
  Top 0.406: U13.4 135.89,60.73 135.89,62.23
  Top 1.016: 135.89,62.23 R11.2
N$21
  Top 0.406: U8.4 97.79,60.73 97.79,62.23
  Top 1.016: 97.79,62.23 R5.2
N$23
  Top 0.406: U9.4 110.49,60.73 110.49,62.23
  Top 1.016: 110.49,62.23 R6.2
N$27
  Top 1.27: JP10.1 13.12,65.62 C27.1 12.88,60.72 IC1.3
  Bottom 1.27: JP9.3 26.67,55.88 25.4,57.15 15.24,57.15 13.97,58.42 13.97,64.77 JP10.1
N$28
  Top 0.406: U6.4 46.99,60.73 46.99,62.23
  Top 1.016: 46.99,62.23 R4.2
N$29
  Top 1.27: IC1.4 IC1.2 12.7,58.42 12.7,57.15 C26.+ 13.13,50.8 JP9.1
N$30
  Top 1.016: X6.1 R5.1
N$31  (1 unrouted)
  Top 1.016: R7.1 59.69,68.58
N$32
  Top 1.016: X7.1 R6.1
N$33
  Top 1.016: X9.1 R8.1
N$34
  Top 1.016: X10.1 R9.1
N$35
  Top 1.016: X12.1 R10.1
N$36
  Top 1.016: X11.1 R11.1
N$37  (via drill 0.6)
  other vias: 24.13,67.95
N$38  (via drill 0.6)
  other vias: 29.21,67.95
N$39  (via drill 0.6)
  other vias: 24.13,65.41
N$40  (via drill 0.6)
  other vias: 25.4,65.41
N$41  (via drill 0.6)
  other vias: 27.94,65.41
N$42  (via drill 0.6)
  other vias: 29.21,65.41
N$43  (via drill 0.6)
  other vias: 29.21,64.14
N$44  (via drill 0.6)
  other vias: 27.94,64.14
N$45  (via drill 0.6)
  other vias: 25.4,64.14
N$46  (via drill 0.6)
  other vias: 24.13,64.14
PPS_OUT_Y1
  Top 0.305: U4.18 15.88,27.3 15.24,26.67 15.24,14.61 8.26,14.61 6.35,12.7 JP4.1
PPS_OUT_Y2
  Top 0.305: U4.17 15.88,28.57 15.24,27.94 13.97,27.94 13.97,21.13 arc-90 13.56,20.72 arc90 13.16,20.31 13.16,19.86 arc90 13.56,19.46 arc-90 13.97,19.05 13.97,17.78 10.15,17.78 arc-90 9.74,18.19 9.74,18.61 arc90 9.34,19.01 7.16,19.01 arc90 6.76,18.61 6.76,18.19 arc-90 6.35,17.78 JP4.3
PPS_OUT_Y3
  Top 0.254: 15.24,29.21 12.7,29.21 12.7,20.96 11.43,20.96 arc-90 11.05,21.34 11.05,22.25 arc90 10.67,22.63 10.28,22.63 arc90 9.9,22.25 9.9,21.34 arc-90 9.52,20.96 6.99,20.96 6.99,22.86 JP5.1
  Top 0.305: U4.16 15.88,29.84 15.24,29.21
PPS_OUT_Y4
  Top 0.305: U4.15 15.88,31.11 15.24,30.48 12.06,30.48 12.06,27.94 11.43,27.94 arc90 11.02,27.53 11.02,27.11 arc-90 10.62,26.7 10.52,26.7 arc-90 10.12,27.11 10.12,28.77 arc90 9.71,29.18 9.62,29.18 arc90 9.21,28.77 9.21,27.11 arc-90 8.8,26.7 8.71,26.7 arc-90 8.3,27.11 8.3,28.77 arc90 7.9,29.18 7.8,29.18 arc90 7.4,28.77 7.4,27.11 arc-90 6.99,26.7 6.9,26.7 arc-90 6.49,27.11 6.49,27.53 arc90 6.08,27.94 JP5.3
PPS_OUT_Y5
  Top 0.305: U4.14 15.88,32.39 15.24,33.02 14.27,33.02 arc-90 13.86,33.43 13.86,33.73 arc90 13.46,34.14 13.25,34.14 arc90 12.85,33.73 12.85,32.31 arc-90 12.44,31.9 12.24,31.9 arc-90 11.83,32.31 11.83,33.73 arc90 11.43,34.14 11.22,34.14 arc90 10.82,33.73 10.82,32.31 arc-90 10.41,31.9 10.21,31.9 arc-90 9.8,32.31 9.8,33.73 arc90 9.39,34.14 9.19,34.14 arc90 8.79,33.73 8.79,32.31 arc-90 8.38,31.9 8.18,31.9 arc-90 7.77,32.31 7.77,33.73 arc90 7.37,34.14 7.16,34.14 arc90 6.76,33.73 6.76,33.43 arc-90 6.35,33.02 JP6.1
PPS_OUT_Y6
  Top 0.254: 15.88,33.66 13.34,36.2 13.34,38.1 9.45,38.1 arc-90 9.07,38.48 9.07,39.63 arc90 8.69,40.01 8.67,40.01 arc90 8.29,39.63 8.29,36.57 arc-90 7.91,36.19 7.89,36.19 arc-90 7.51,36.57 7.51,39.63 arc90 7.13,40.01 7.11,40.01 arc90 6.73,39.63 6.73,38.48 arc-90 6.35,38.1 JP6.3
  Top 0.305: U4.13 15.88,33.66
PPS_OUT_Y7
  Top 0.305: U4.12 15.88,34.92 13.97,36.83 13.97,43.18 10.87,43.18 arc-90 10.46,43.59 10.46,46.11 arc90 10.05,46.52 8.43,46.52 arc90 8.03,46.11 8.03,43.59 arc-90 7.62,43.18 JP7.1
PPS_OUT_Y8
  Top 0.305: U4.11 15.88,36.2 15.24,36.83 15.24,46.99 13.97,48.26 9.47,48.26 arc-90 9.06,48.67 9.06,49.29 arc90 8.66,49.69 8.43,49.69 arc90 8.03,49.29 8.03,48.67 arc-90 7.62,48.26 JP7.3
VCC_10MHZ  (via drill 0.6)  (1 unrouted)
  Top 0.406: C10.2 44.03,61.59 45.72,61.59 45.72,60.73 U6.5 | C12.2 56.73,61.59 58.42,61.59 58.42,60.73 U7.5 | C18.2 69.43,61.59 71.12,61.59 71.12,60.73 U10.5 | C20.2 82.13,61.59 83.82,61.59 83.82,60.73 U11.5 | C14.2 94.83,61.59 96.52,61.59 96.52,60.73 U8.5 | C16.2 107.53,61.59 109.22,61.59 109.22,60.73 U9.5 | C22.2 120.23,61.59 121.92,61.59 121.92,60.73 U12.5 | C24.2 132.93,61.59 134.62,61.59 134.62,60.73 U13.5
  Top 0.61: U5.5 89.53,11.2 89.53,10.79 87,10.79 C8.2 C7.2
  Top 0.813: 44.45,62.23 43.81,62.23 43.81,59.69 C9.2 | 56.73,61.59 56.52,61.59 56.52,59.69 C11.2 | 69.43,61.59 69.22,61.59 69.22,59.69 C17.2 | 82.13,61.59 81.92,61.59 81.92,59.69 C19.2 | 94.83,61.59 94.61,61.59 94.61,59.69 C13.2 | 107.53,61.59 107.31,61.59 107.31,59.69 C15.2 | 120.23,61.59 120.02,61.59 120.02,59.69 C21.2 | 132.93,61.59 132.72,61.59 132.72,59.69 C23.2
  Top 1.27: v44.45,64.77 44.45,62.23 | C12.2 57.15,62.23 v57.15,64.77 | C18.2 69.85,62.23 v69.85,64.77 | C20.2 82.55,62.23 v82.55,64.77 | C14.2 95.25,62.23 v95.25,64.77 | C16.2 107.95,62.23 v107.95,64.77 | C22.2 120.65,62.23 v120.65,64.77 | C24.2 133.35,62.23 v133.35,64.77 | 87,10.79 v81.92,10.79
  Bottom 1.27: 39.37,50.8 39.37,64.77 v44.45,64.77 v57.15,64.77 v69.85,64.77 v82.55,64.77 v95.25,64.77 v107.95,64.77 v120.65,64.77 v133.35,64.77 | v81.92,10.79 39.37,50.8 | 39.37,50.8 JP8.2
(copper drawn outside any net)
  shapes: Bottom area x2, Top area x2

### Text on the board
tNames: + VCC | +3.3V | - VSS | Clock CMOS/TTL outputs | 1PPS OUT | < Clock level | 5V SOURCE > | 1-2 TTL | 2-3 CMOS | 1-2 INT REG | 2-3 EXTERNAL | +5V | 1PPS CMOS outputs | phases matching | U4 outputs control | JP3 OE1 | JP2 OE2 | 1-2 HIGH Z | 2-3 LOW | P G P G P G P G P G P G P G P G | ALL INPUTS 5.5 V MAX | CMOS 1PPS distribution 1:8 | CMOS/TTL Clock distribution 1:8 | 1PPS CTRL | Square wave clock input > | Oleg Kutkov, 2021 | 1PPS OUT 5V > | 1PPS IN > | 1MHz - 40MHz, CMOS/TTL | https://olegkutkov.me

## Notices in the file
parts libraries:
SparkFun-Connectors: Licensing: Creative Commons ShareAlike 4.0 International - https://creativecommons.org/licenses/by-sa/4.0
